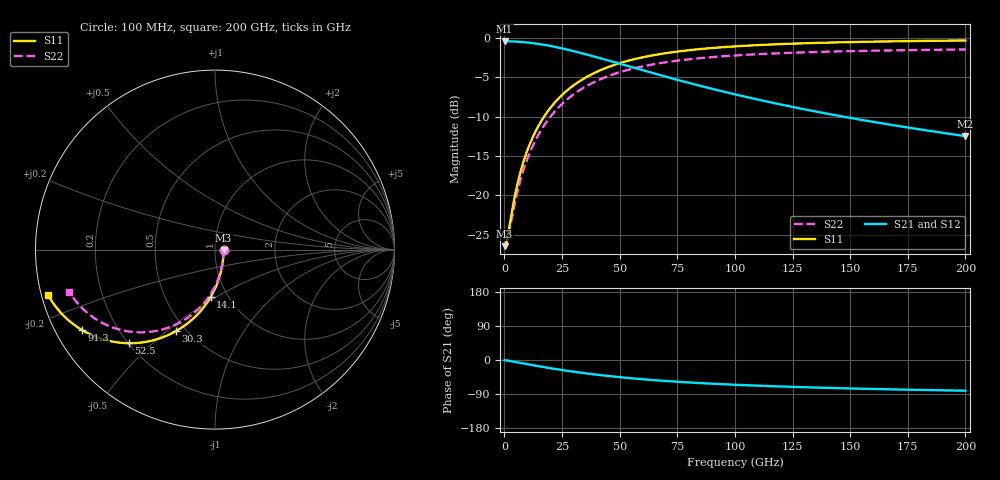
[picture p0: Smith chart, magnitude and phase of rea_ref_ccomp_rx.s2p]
! Created with skrf 1.10.0 (http://scikit-rf.org).
# Hz S RI R 50.0
!freq ReS11 ImS11 ReS21 ImS21 ReS12 ImS12 ReS22 ImS22
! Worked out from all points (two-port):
!   2000 points, 100 MHz to 200 GHz, reference 50 ohm
!   highest |S21| = -0.42 dB at 100 MHz (marker M1); lowest = -12.5 dB at 200 GHz (marker M2)
!   |S21| within 3 dB of the highest: start of sweep to 51.77 GHz
!   lowest |S11| = -26.4 dB at 100 MHz (marker M3), VSWR 1.10, Z = 55 - j0.221 ohm
!   |S11| at or under -10 dB: start of sweep to 17.2 GHz
!   |S22| runs from -26.4 to -1.5 dB; largest |S21 - S12| = 1.2e-16
!   S11 on the Smith chart (normalised r, x): 100 MHz: 1.10, -0.00; 14.1 GHz: 0.83, -0.47; 30.3 GHz: 0.44, -0.54; 52.5 GHz: 0.20, -0.42; 91.3 GHz: 0.08, -0.28; 200 GHz: 0.02, -0.13
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1e8  0.0476 -0.00201  0.9524 -0.00188  0.9524 -0.00188  0.0476 -0.00177
8e8  0.0474 -0.0161  0.9521 -0.015  0.9521 -0.015  0.0474 -0.0142
1.6e9  0.0466 -0.0321  0.9515 -0.0301  0.9515 -0.0301  0.0468 -0.0283
4.7e9  0.0391 -0.0937  0.9444 -0.0877  0.9444 -0.0877  0.0402 -0.0825
7.3e9  0.0274 -0.1438  0.9334 -0.1346  0.9334 -0.1346  0.0299 -0.1267
1.04e10  0.00739 -0.2009  0.9147 -0.188  0.9147 -0.188  0.0123 -0.177
1.41e10  -0.024 -0.2638  0.8853 -0.247  0.8853 -0.247  -0.0153 -0.2324
1.75e10  -0.0588 -0.3157  0.8527 -0.2955  0.8527 -0.2955  -0.0458 -0.2782
2.13e10  -0.1026 -0.3663  0.8116 -0.3428  0.8116 -0.3428  -0.0843 -0.3228
2.56e10  -0.1563 -0.4137  0.7613 -0.3872  0.7613 -0.3872  -0.1314 -0.3647
3.03e10  -0.2173 -0.4541  0.7042 -0.425  0.7042 -0.425  -0.185 -0.4005
3.35e10  -0.2589 -0.4752  0.6652 -0.4447  0.6652 -0.4447  -0.2215 -0.4192
4.23e10  -0.3684 -0.5108  0.5626 -0.478  0.5626 -0.478  -0.3176 -0.451
5.25e10  -0.4796 -0.5216  0.4584 -0.4879  0.4584 -0.4879  -0.4153 -0.4611
6.68e10  -0.6025 -0.5055  0.3433 -0.4727  0.3433 -0.4727  -0.5232 -0.4479
7.85e10  -0.6779 -0.4801  0.2727 -0.4487  0.2727 -0.4487  -0.5894 -0.4263
9.13e10  -0.7405 -0.4484  0.2141 -0.4188  0.2141 -0.4188  -0.6444 -0.3993
1.001e11  -0.7742 -0.4265  0.1825 -0.3982  0.1825 -0.3982  -0.6741 -0.3806
1.156e11  -0.8203 -0.3901  0.1394 -0.3638  0.1394 -0.3638  -0.7146 -0.3496
1.334e11  -0.8582 -0.3528  0.1039 -0.3287  0.1039 -0.3287  -0.748 -0.318
1.667e11  -0.9032 -0.2965  0.0618 -0.2754  0.0618 -0.2754  -0.7878 -0.2706
2e11  -0.9295 -0.2541  0.0372 -0.2353  0.0372 -0.2353  -0.8113 -0.2354
